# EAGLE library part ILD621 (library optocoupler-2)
SIEMENS OPTO COUPLER
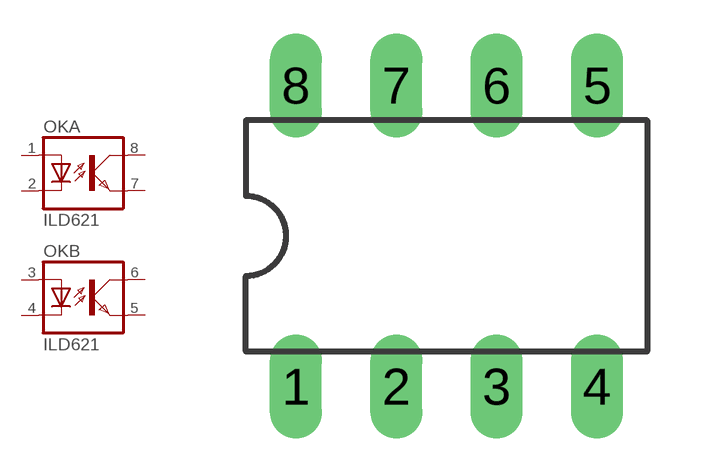
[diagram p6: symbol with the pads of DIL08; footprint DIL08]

Designator prefix OK; gates A=OK B=OK

## ILD621  [DIL08]
1  A:A  pas
2  A:C  pas
3  B:A  pas
4  B:C  pas
5  B:EMIT  pas
6  B:COL  pas
7  A:EMIT  pas
8  A:COL  pas

## Footprint DIL08 (pad centres in mm)
Dual In Line Package
drill 0.813 long: 1 -3.81,-3.81; 2 -1.27,-3.81; 3 1.27,-3.81; 4 3.81,-3.81; 5 3.81,3.81; 6 1.27,3.81; 7 -1.27,3.81; 8 -3.81,3.81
